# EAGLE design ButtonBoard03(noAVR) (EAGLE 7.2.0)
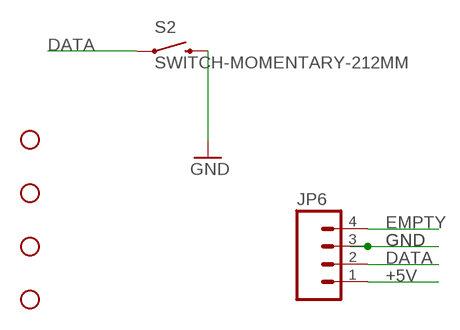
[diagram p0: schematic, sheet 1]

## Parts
JP2  STAND-OFF  [STAND-OFF]
JP3  STAND-OFF  [STAND-OFF]
JP4  STAND-OFF  [STAND-OFF]
JP5  STAND-OFF  [STAND-OFF]
JP6  M04LONGPADS  [1X04_LONGPADS]
S2  SWITCH-MOMENTARY-212MM  [TACTILE-PTH-12MM]

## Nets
+5V: JP6.1
DATA: JP6.2 S2.1
EMPTY: JP6.4
GND: JP6.3 S2.3

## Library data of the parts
JP2-JP5 = 01_SparkFun:STAND-OFF: Stand Off
JP6 = 01_SparkFun:M04: Header 4 Standard 4-pin 0.1" header. Use with straight break away headers (SKU : PRT-00116), right angle break away headers (PRT-00553), swiss pins (PRT-00743), machine pins (PRT-00117), and female headers (PRT-00115). Molex polarized connector foot print use with SKU : PRT-08231 with associated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
S2 = SparkFun-Electromechanical:SWITCH-MOMENTARY-2: Various NO switches- pushbuttons, reed, etc

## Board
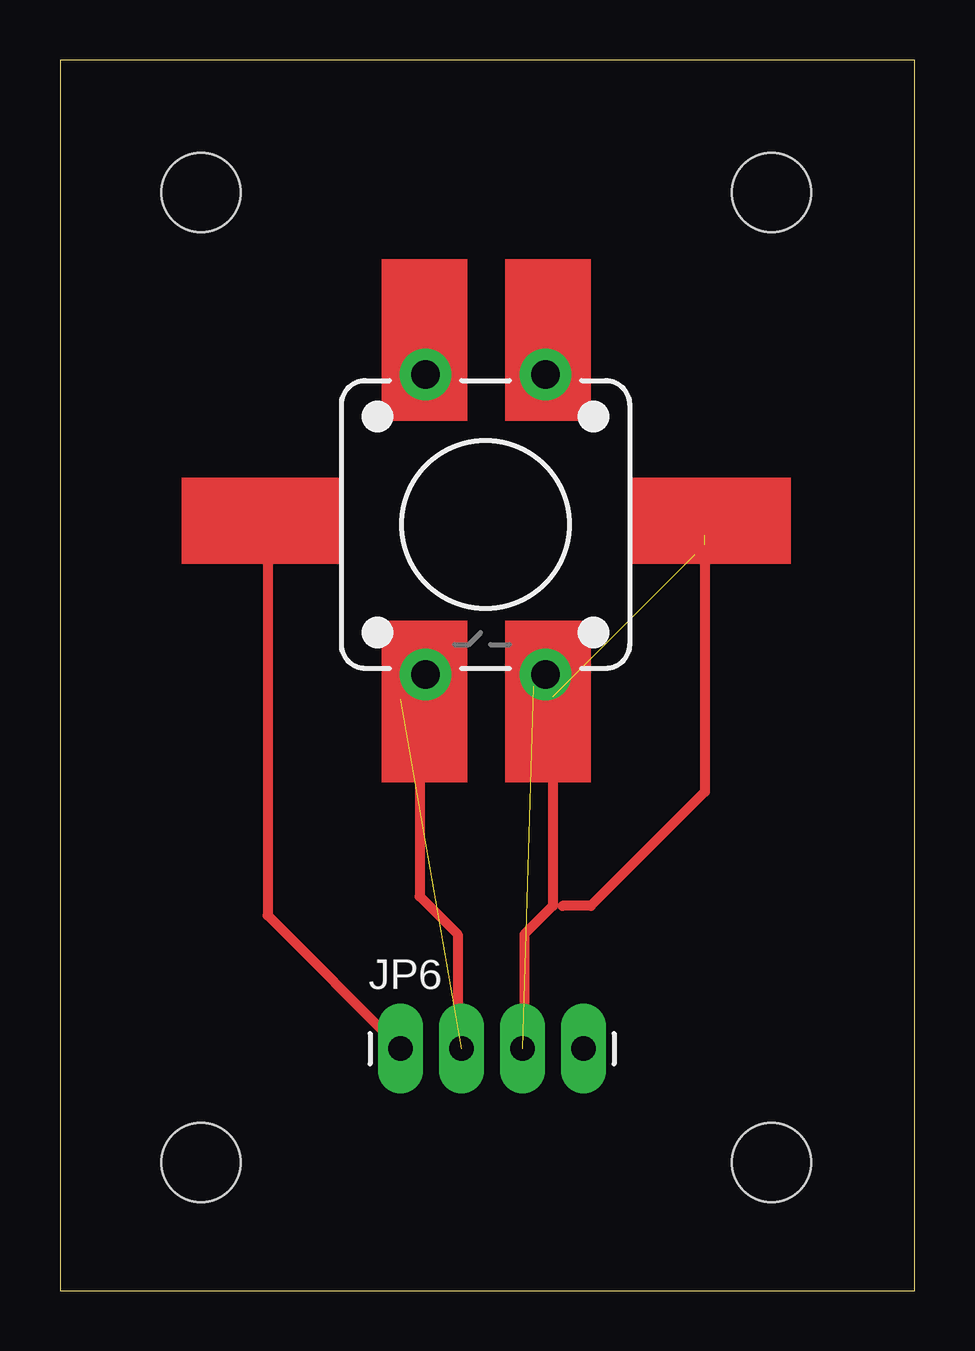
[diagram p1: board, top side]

Size 35.62 x 51.28 mm. Coordinates in mm from the lower left corner, seen from the top.
Outline: 0,0 35.62,0 35.62,51.28 0,51.28 0,0
Copper layers (1*16): Top 0.035mm / dielectric 1.5mm / Bottom 0.035mm
Design rules "default": minimum track width 10mil, minimum drill 24mil, track to track 8mil, track to pad 8mil, pad to pad 8mil, via to via 8mil, smd to smd 8mil, copper to edge 40mil, drill to drill 8mil, minimum pad ring 10mil, minimum via ring 8mil, stop-mask expansion 4mil, vias tented up to drill 0mil, thermal gap 10mil

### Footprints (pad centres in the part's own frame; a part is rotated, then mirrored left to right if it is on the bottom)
STAND-OFF = hole 3.302: 0,0
1X04_LONGPADS = drill 1.016 pad 1.88 long: 1 0,0; 2 2.54,0; 3 5.08,0; 4 7.62,0
TACTILE-PTH-12MM = drill 1.2 pad 2.159: 1 6.25,-2.5; 2 -6.25,-2.5; 3 6.25,2.5; 4 -6.25,2.5

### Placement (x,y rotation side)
JP2  5.87,5.33 0 top
JP3  29.65,5.33 0 top
JP4  29.65,45.75 0 top
JP5  5.87,45.75 0 top
JP6  14.19,10.09 0 top
S2  17.73,31.92 270 top

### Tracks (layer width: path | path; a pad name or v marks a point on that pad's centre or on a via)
+5V
  Top 0.406: 8.65,31.49 8.65,15.64 JP6.1
DATA  (1 unrouted)
  Top 0.406: S2.1 14.19,24.64
GND  (1 unrouted)
  Top 0.406: S2.3 19.74,25.18
N$1
  Top 0.406: 26.87,31.88 26.87,20.79 22.12,16.03 20.93,16.03
N$3  (2 unrouted)
  Top 0.406: 26.87,31.49 26.48,31.09 | 20.14,25.15 20.53,24.75 20.53,16.03 19.34,14.84 19.34,8.9 | 26.87,31.09 26.48,30.69
N$4
  Top 0.406: 15.38,25.54 14.99,25.15 14.99,16.43 16.57,14.84 16.57,10.09
(copper drawn outside any net)
  shapes: Top area x6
